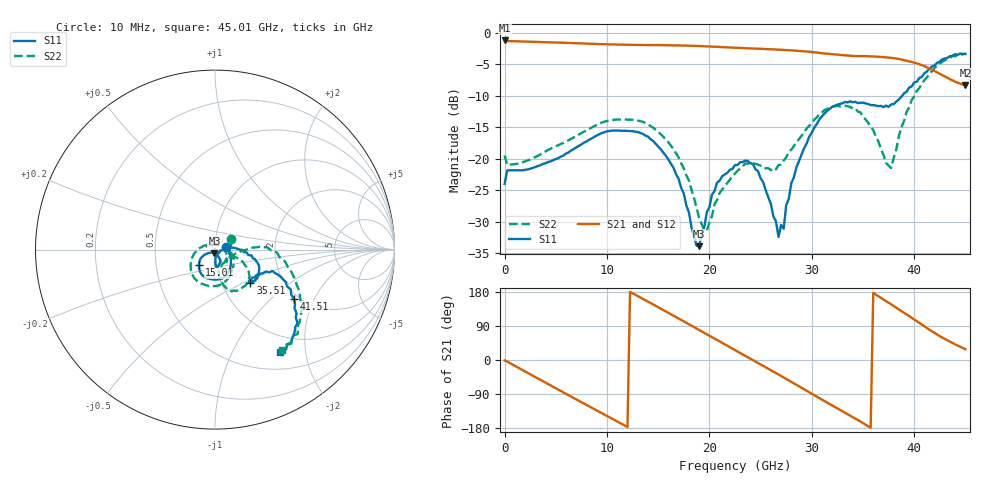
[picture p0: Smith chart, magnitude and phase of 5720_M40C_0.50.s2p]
! Device:  ADRF5720
! Description: 0.5dB LSB GaAs MMIC 6-bit Digital Attenuator
! Frequency:  0.000009 -  40 GHz
! Ports:
!	RF1	= Port 1
!	RF2	= Port 2
! Vdd:  3.3 Volt
! Vss:  -3.3 Volt
! Control:  0/3.3 Volt
! State:  0.50 dB attenuation
! Data:  The device was measured using G-S-G Probes on a matrix board.
!  Data was collected using an calibrated 4 port network analyzer.
!  The reference plane for this measurement is at the launchers.
! Note:  Analog Devices supplies this data as a sample of measured data
!  for this product.  Your particular data for this product may vary.
!  Data was taken at -40 degrees C.
!  Analog Devices reserves the right to change this data at anytime.
# GHZ S DB R 45.0
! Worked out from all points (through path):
!   181 points, 10 MHz to 45.01 GHz, reference 45 ohm
!   highest |S21| = -1.25 dB at 10 MHz (marker M1); lowest = -8.3 dB at 45.01 GHz (marker M2)
!   group delay of S21, straight-line fit = 42.6 ps
!   lowest |S11| = -33.9 dB at 19.01 GHz (marker M3), VSWR 1.04, Z = 44.7 - j1.79 ohm
!   |S11| at or under -10 dB: start of sweep to 38.84 GHz
!   |S22| runs from -31.4 to -3.4 dB; largest |S21 - S12| = 0.0031
!   S11 on the Smith chart (normalised r, x): 10 MHz: 1.13, +0.03; 15.01 GHz: 0.82, -0.15; 35.51 GHz: 1.36, -0.55; 41.51 GHz: 1.87, -1.41; 45.01 GHz: 0.74, -1.56
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0.01  -23.99 13.1  -1.25 -1.2  -1.27 -1.2  -19.47 33.2
2.01  -21.76 -14.3  -1.43 -30.3  -1.45 -30.3  -20.42 -14.5
4.26  -20.51 -22.4  -1.54 -63.5  -1.56 -63.5  -18.60 -27.3
7.76  -17.44 -51.1  -1.73 -114.9  -1.75 -115.0  -15.68 -58.5
11.51  -15.57 -92.6  -1.92 -169.4  -1.94 -169.5  -13.77 -100.8
15.01  -18.07 -135.8  -1.99 139.3  -2.00 139.2  -15.76 -146.4
15.26  -18.49 -138.5  -1.99 135.5  -2.01 135.5  -16.11 -150.0
17.51  -25.52 -152.9  -2.06 101.9  -2.08 101.8  -21.53 173.2
19.01  -33.85 -98.7  -2.13 79.2  -2.15 79.1  -29.37 123.5
19.76  -28.44 -67.8  -2.18 67.9  -2.20 67.8  -31.42 61.9
20.76  -23.75 -62.9  -2.26 52.8  -2.28 52.7  -26.54 6.7
22.76  -20.98 -78.5  -2.42 22.7  -2.44 22.6  -21.90 -32.7
24.76  -21.97 -88.5  -2.56 -7.5  -2.57 -7.6  -20.92 -46.8
26.76  -32.39 -50.9  -2.71 -38.2  -2.73 -38.4  -20.97 -28.9
28.51  -21.33 7.5  -2.88 -65.5  -2.90 -65.7  -17.43 -20.7
30.26  -15.05 -5.2  -3.12 -93.1  -3.15 -93.2  -13.78 -29.7
33.26  -10.99 -29.7  -3.61 -139.3  -3.64 -139.5  -11.60 -58.4
35.51  -11.33 -43.3  -3.75 -174.7  -3.78 -174.9  -14.29 -77.3
37.76  -11.38 -35.0  -4.01 146.9  -4.04 146.7  -21.47 -36.1
39.26  -9.39 -20.4  -4.47 120.2  -4.49 120.1  -12.59 3.3
41.51  -5.71 -32.1  -5.71 79.7  -5.73 79.5  -6.50 -20.2
45.01  -3.38 -57.6  -8.33 28.5  -8.35 28.4  -3.40 -56.2
